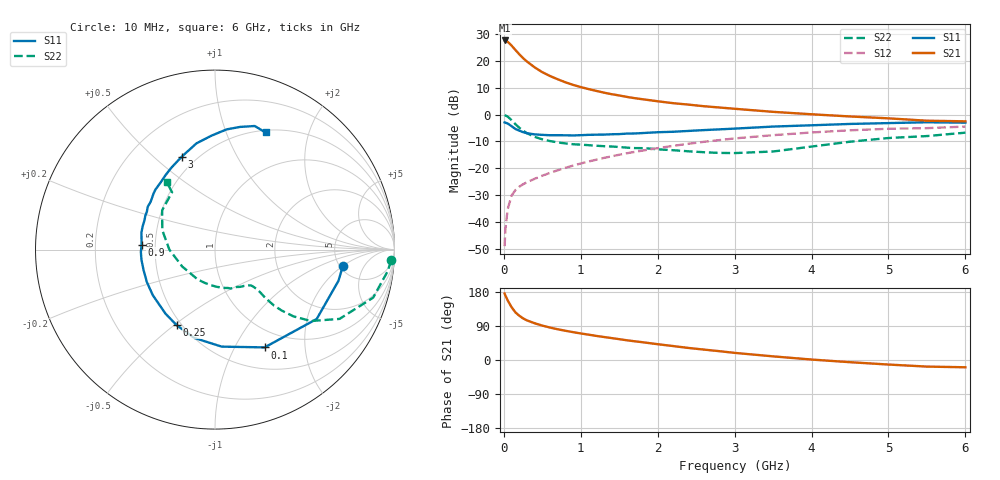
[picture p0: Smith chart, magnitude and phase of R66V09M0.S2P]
! SIEMENS Small Signal Semiconductors
! BFR193
! Si NPN RF Bipolar Junction Transistor in SOT23
! VCE = 6 V  IC = 9 mA
! Common Emitter S-Parameters:  May  1996
# GHz  S  MA  R  50
!  f  S11  S21  S12  S22
! GHz  MAG  ANG  MAG  ANG  MAG  ANG  MAG  ANG
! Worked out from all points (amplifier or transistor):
!   36 points, 10 MHz to 6 GHz, reference 50 ohm
!   highest |S21| = 27.8 dB at 10 MHz (marker M1)
!   |S21| within 3 dB of that: start of sweep to 133.4 MHz
!   unconditionally stable (mu >= 1): 773.1 MHz to 1.939 GHz
!   at 250 MHz: K = 0.60, MSG = 23.6 dB, |S12| = -26.0 dB
!   at 1.4 GHz: K = 1.04, MAG = 10.4 dB, |S12| = -15.6 dB
!   at 6 GHz: K = 0.94, MSG = 1.0 dB, |S12| = -4.4 dB
!   S11 on the Smith chart (normalised r, x): 10 MHz: 5.34, -1.99; 100 MHz: 0.76, -1.33; 250 MHz: 0.47, -0.51; 900 MHz: 0.42, +0.03; 3 GHz: 0.42, +0.62; 6 GHz: 0.53, +1.39
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0.01  0.7184 -7.2  24.42 175.3  0.0035 85.5  0.9831 -3.5
0.02  0.7095 -14.2  24.41 170.3  0.0072 81.9  0.9699 -7.1
0.05  0.686 -34.3  23.07 157.3  0.0172 74.6  0.9209 -16.9
0.1  0.611 -63.1  19.62 139.5  0.0307 64.6  0.7939 -29.1
0.15  0.5418 -86.1  16.24 125.8  0.039 57.9  0.6657 -36.7
0.2  0.5054 -103.3  13.52 116.9  0.0451 55.6  0.5738 -40.4
0.25  0.4724 -116.8  11.41 109.8  0.0502 54.5  0.504 -42.4
0.3  0.451 -127.7  9.866 104.5  0.0546 55.1  0.4523 -43.5
0.4  0.4297 -143.7  7.69 97.0  0.0635 56.6  0.3858 -43.8
0.5  0.4206 -154.5  6.235 90.8  0.0726 57.8  0.3472 -43.4
0.6  0.4139 -164.2  5.289 85.6  0.082 59.5  0.3224 -43.4
0.7  0.4137 -172.2  4.599 81.1  0.0917 60.7  0.3044 -43.8
0.9  0.4102 176.3  3.612 73.5  0.1121 61.9  0.2811 -45.1
1.1  0.421 166.7  3.018 66.9  0.1336 62.1  0.27 -48.2
1.3  0.4252 157.6  2.59 60.7  0.156 61.7  0.2584 -51.6
1.6  0.4445 147.4  2.151 52.0  0.1906 60.3  0.2426 -59.1
2.2  0.4806 129.3  1.644 36.8  0.2622 55.0  0.2172 -78.7
3  0.5503 109.6  1.292 18.8  0.3607 44.8  0.1921 -120.5
3.5  0.6008 99.9  1.132 9.6  0.415 37.4  0.2056 -152.8
4.5  0.6728 84.5  0.928 -5.8  0.5119 22.4  0.3133 159.7
5.5  0.7232 72.2  0.773 -17.4  0.5614 6.7  0.3993 126.8
6  0.7109 66.6  0.753 -19.2  0.6007 2.2  0.4621 125.6
